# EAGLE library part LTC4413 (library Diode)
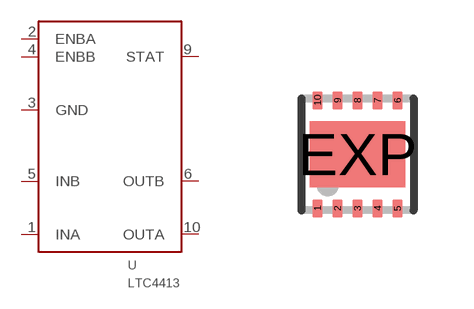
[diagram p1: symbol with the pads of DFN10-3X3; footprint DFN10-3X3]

Designator prefix U

## LTC4413  [DFN10-3X3]
1  INA
2  ENBA
3  GND
4  ENBB
5  INB
6  OUTB
9  STAT
10  OUTA
EXP  THERMAL_PAD

## Footprint DFN10-3X3 (pad centres in mm)
DD Package 10-Lead Plastic DFN (3mm × 3mm) (Reference LTC DWG # 05-08-1669) Source: http://www.linear.com .. 4062fa.pdf
smd 0.25 x 0.45: 1 -1,-1.35; 2 -0.5,-1.35; 3 0,-1.35; 4 0.5,-1.35; 5 1,-1.35; 6 1,1.35; 7 0.5,1.35; 8 0,1.35; 9 -0.5,1.35; 10 -1,1.35
smd 2.38 x 1.65: EXP 0,0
